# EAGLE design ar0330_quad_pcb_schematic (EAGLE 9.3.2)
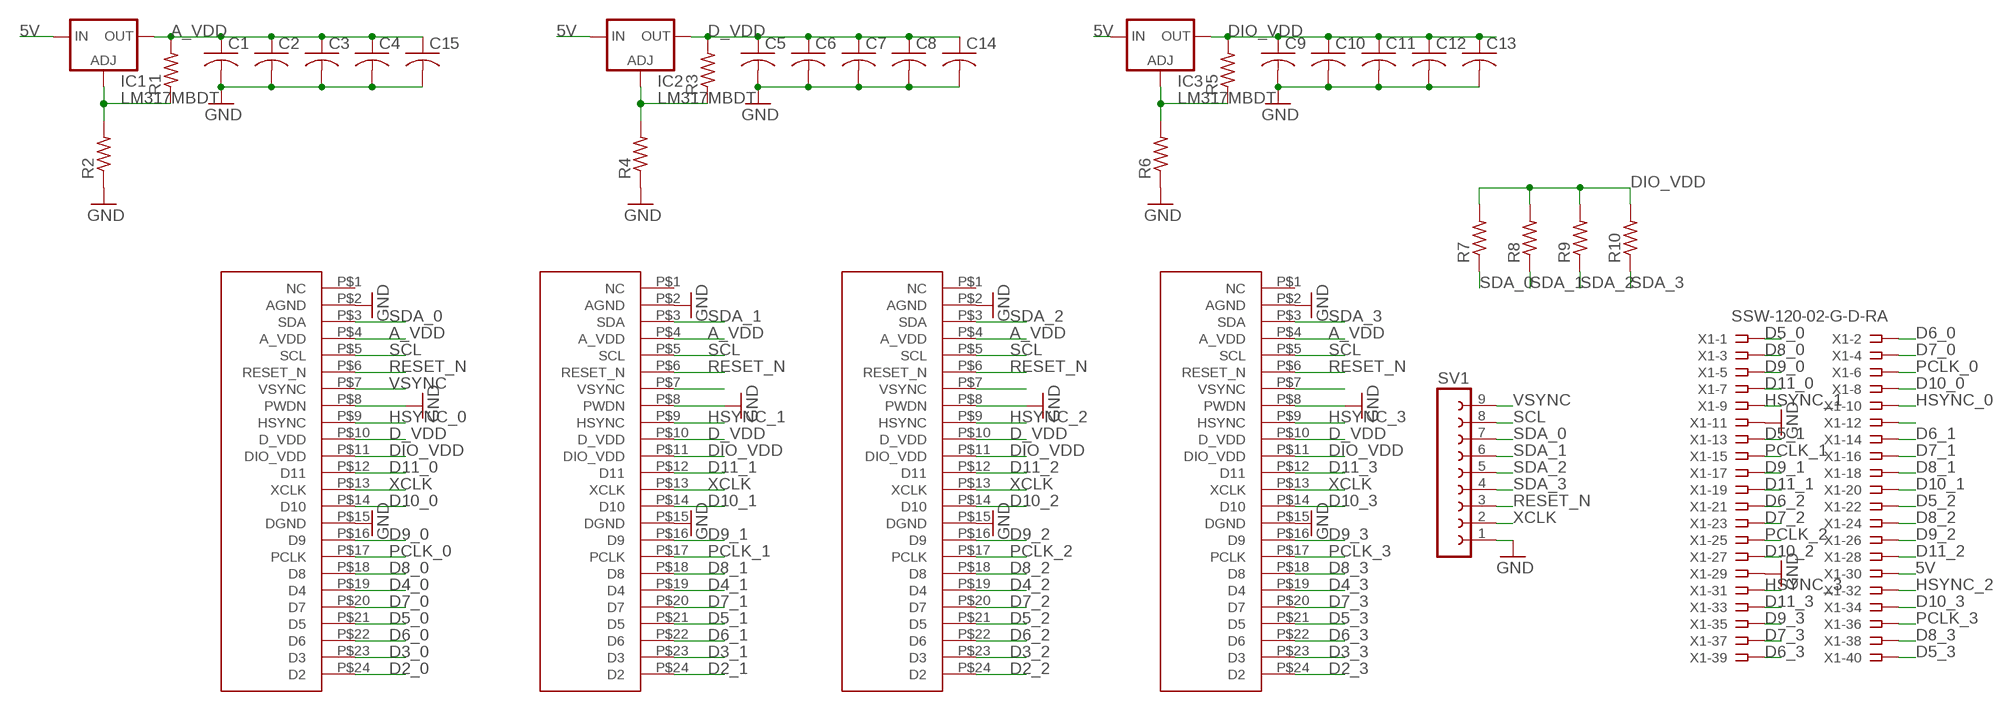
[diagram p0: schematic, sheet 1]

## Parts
C1  C-USC0805  [C0805]
C2  C-USC0805  [C0805]
C3  C-USC0805  [C0805]
C4  C-USC0805  [C0805]
C5  C-USC0805  [C0805]
C6  C-USC0805  [C0805]
C7  C-USC0805  [C0805]
C8  C-USC0805  [C0805]
C9  C-USC0805  [C0805]
C10  C-USC0805  [C0805]
C11  C-USC0805  [C0805]
C12  C-USC0805  [C0805]
C13  C-USC0805  [C0805]
C14  C-USC0805  [C0805]
C15  C-USC0805  [C0805]
IC1  LM317MBDT  [DPACK]
IC2  LM317MBDT  [DPACK]
IC3  LM317MBDT  [DPACK]
R1  R-US_R0805  [R0805]
R2  R-US_R0805  [R0805]
R3  R-US_R0805  [R0805]
R4  R-US_R0805  [R0805]
R5  R-US_R0805  [R0805]
R6  R-US_R0805  [R0805]
R7  R-US_R0805  [R0805]
R8  R-US_R0805  [R0805]
R9  R-US_R0805  [R0805]
R10  R-US_R0805  [R0805]
SV1  FE09-1  [FE09]
U$1  AR0330_FPC_24  [FPC_24_0P5]
U$2  AR0330_FPC_24  [FPC_24_0P5]
U$3  AR0330_FPC_24  [FPC_24_0P5]
U$4  AR0330_FPC_24  [FPC_24_0P5]
X1  SSW-120-02-G-D-RA  [SSW-120-02-G-D-RA]

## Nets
5V: IC1.3(IN) IC2.3(IN) IC3.3(IN) X1.30
A_VDD: C1.1 C2.1 C3.1 C4.1 C15.1 IC1.4(OUT) R1.2 U$1.P$4(A_VDD) U$2.P$4(A_VDD) U$3.P$4(A_VDD) U$4.P$4(A_VDD)
D2_0: U$1.P$24(D2)
D2_1: U$2.P$24(D2)
D2_2: U$3.P$24(D2)
D2_3: U$4.P$24(D2)
D3_0: U$1.P$23(D3)
D3_1: U$2.P$23(D3)
D3_2: U$3.P$23(D3)
D3_3: U$4.P$23(D3)
D4_0: U$1.P$19(D4)
D4_1: U$2.P$19(D4)
D4_2: U$3.P$19(D4)
D4_3: U$4.P$19(D4)
D5_0: U$1.P$21(D5) X1.1
D5_1: U$2.P$21(D5) X1.13
D5_2: U$3.P$21(D5) X1.22
D5_3: U$4.P$21(D5) X1.40
D6_0: U$1.P$22(D6) X1.2
D6_1: U$2.P$22(D6) X1.14
D6_2: U$3.P$22(D6) X1.21
D6_3: U$4.P$22(D6) X1.39
D7_0: U$1.P$20(D7) X1.4
D7_1: U$2.P$20(D7) X1.16
D7_2: U$3.P$20(D7) X1.23
D7_3: U$4.P$20(D7) X1.37
D8_0: U$1.P$18(D8) X1.3
D8_1: U$2.P$18(D8) X1.18
D8_2: U$3.P$18(D8) X1.24
D8_3: U$4.P$18(D8) X1.38
D9_0: U$1.P$16(D9) X1.5
D9_1: U$2.P$16(D9) X1.17
D9_2: U$3.P$16(D9) X1.26
D9_3: U$4.P$16(D9) X1.35
D10_0: U$1.P$14(D10) X1.8
D10_1: U$2.P$14(D10) X1.20
D10_2: U$3.P$14(D10) X1.27
D10_3: U$4.P$14(D10) X1.34
D11_0: U$1.P$12(D11) X1.7
D11_1: U$2.P$12(D11) X1.19
D11_2: U$3.P$12(D11) X1.28
D11_3: U$4.P$12(D11) X1.33
D_VDD: C5.1 C6.1 C7.1 C8.1 C14.1 IC2.4(OUT) R3.2 U$1.P$10(D_VDD) U$2.P$10(D_VDD) U$3.P$10(D_VDD) U$4.P$10(D_VDD)
DIO_VDD: C9.1 C10.1 C11.1 C12.1 C13.1 IC3.4(OUT) R5.2 R7.2 R8.2 R9.2 R10.2 U$1.P$11(DIO_VDD) U$2.P$11(DIO_VDD) U$3.P$11(DIO_VDD) U$4.P$11(DIO_VDD)
GND: C1.2 C2.2 C3.2 C4.2 C5.2 C6.2 C7.2 C8.2 C9.2 C10.2 C11.2 C12.2 C13.2 C14.2 C15.2 R2.1 R4.1 R6.1 SV1.1 U$1.P$2(AGND) U$1.P$8(PWDN) U$1.P$15(DGND) U$2.P$2(AGND) U$2.P$8(PWDN) U$2.P$15(DGND) U$3.P$2(AGND) U$3.P$8(PWDN) U$3.P$15(DGND) U$4.P$2(AGND) U$4.P$8(PWDN) U$4.P$15(DGND) X1.11 X1.29
HSYNC_0: U$1.P$9(HSYNC) X1.10
HSYNC_1: U$2.P$9(HSYNC) X1.9
HSYNC_2: U$3.P$9(HSYNC) X1.32
HSYNC_3: U$4.P$9(HSYNC) X1.31
N$16: U$2.P$7(VSYNC)
N$31: U$3.P$7(VSYNC)
N$37: X1.12
N$46: U$4.P$7(VSYNC)
N$63: IC1.1(ADJ) R1.1 R2.2
N$64: IC2.1(ADJ) R3.1 R4.2
N$66: IC3.1(ADJ) R5.1 R6.2
PCLK_0: U$1.P$17(PCLK) X1.6
PCLK_1: U$2.P$17(PCLK) X1.15
PCLK_2: U$3.P$17(PCLK) X1.25
PCLK_3: U$4.P$17(PCLK) X1.36
RESET_N: SV1.3 U$1.P$6(RESET_N) U$2.P$6(RESET_N) U$3.P$6(RESET_N) U$4.P$6(RESET_N)
SCL: SV1.8 U$1.P$5(SCL) U$2.P$5(SCL) U$3.P$5(SCL) U$4.P$5(SCL)
SDA_0: R7.1 SV1.7 U$1.P$3(SDA)
SDA_1: R8.1 SV1.6 U$2.P$3(SDA)
SDA_2: R9.1 SV1.5 U$3.P$3(SDA)
SDA_3: R10.1 SV1.4 U$4.P$3(SDA)
VSYNC: SV1.9 U$1.P$7(VSYNC)
XCLK: SV1.2 U$1.P$13(XCLK) U$2.P$13(XCLK) U$3.P$13(XCLK) U$4.P$13(XCLK)
Unconnected: U$1.P$1(NC) U$2.P$1(NC) U$3.P$1(NC) U$4.P$1(NC)

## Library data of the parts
C1-C15 = rcl:C-US: CAPACITOR, American symbol; SPICEPREFIX: C
IC1-IC3 = v-reg:LM317?*: 500 mA Adjustable Output Positive Voltage Regulator Source: http://www.onsemi.co.jp .. LM317M-D.PDF
R1-R10 = rcl:R-US_: RESISTOR, American symbol; SPICEPREFIX: R
SV1 = con-lsta:FE09-1: FEMALE HEADER; OC_FARNELL: unknown; OC_NEWARK: unknown
U$1-U$4 = FPC_24_0P5:AR0330_FPC_24
X1 = con-samtec:SSW-120-02-G: THROUGH-HOLE .025" SQ POST SOCKET Source: Samtec SSW.pdf; MF: Samtec Inc.; MPN: SSW-120-02-G-D-RA; OC_FARNELL: unknown; OC_NEWARK: 11P9640

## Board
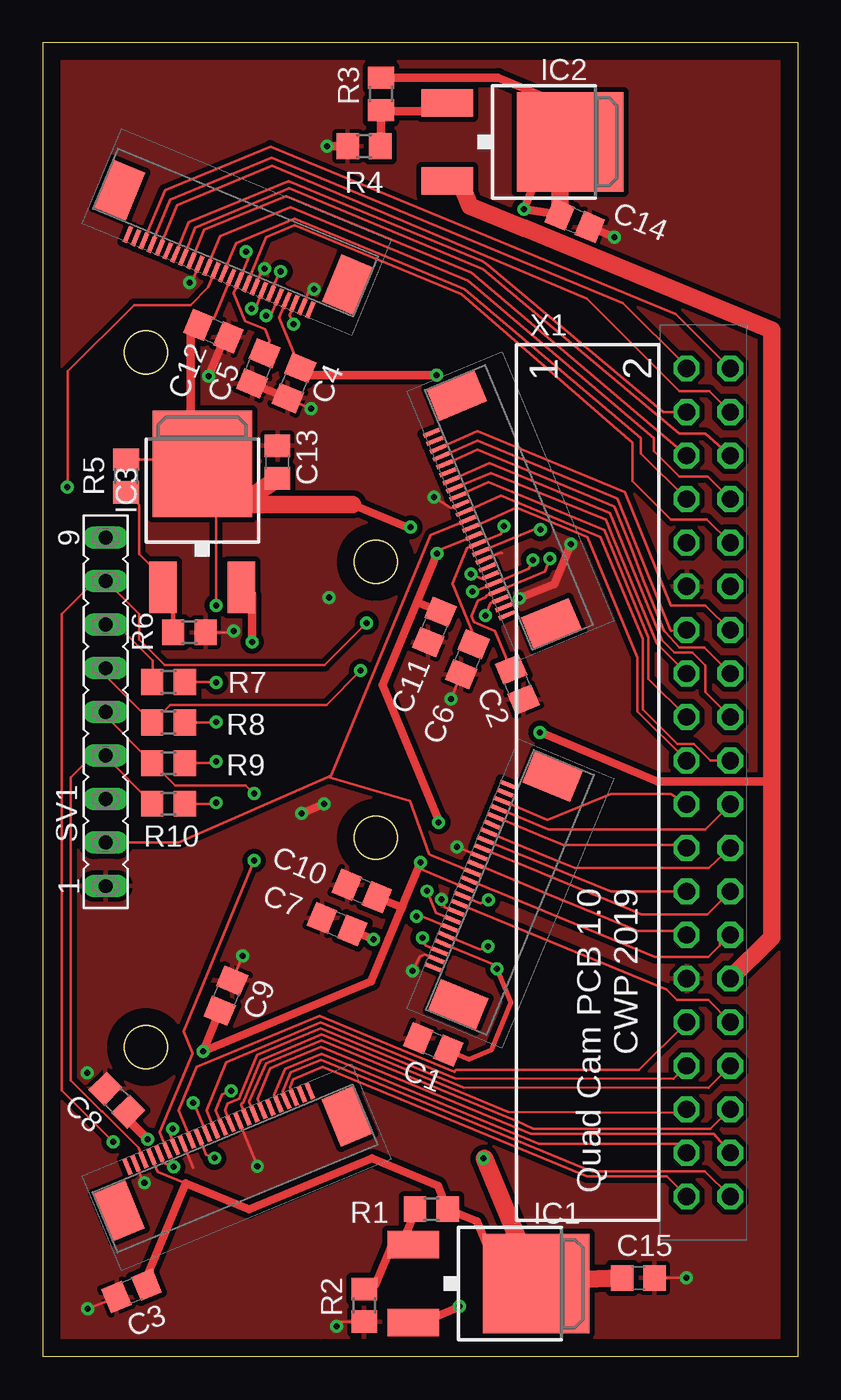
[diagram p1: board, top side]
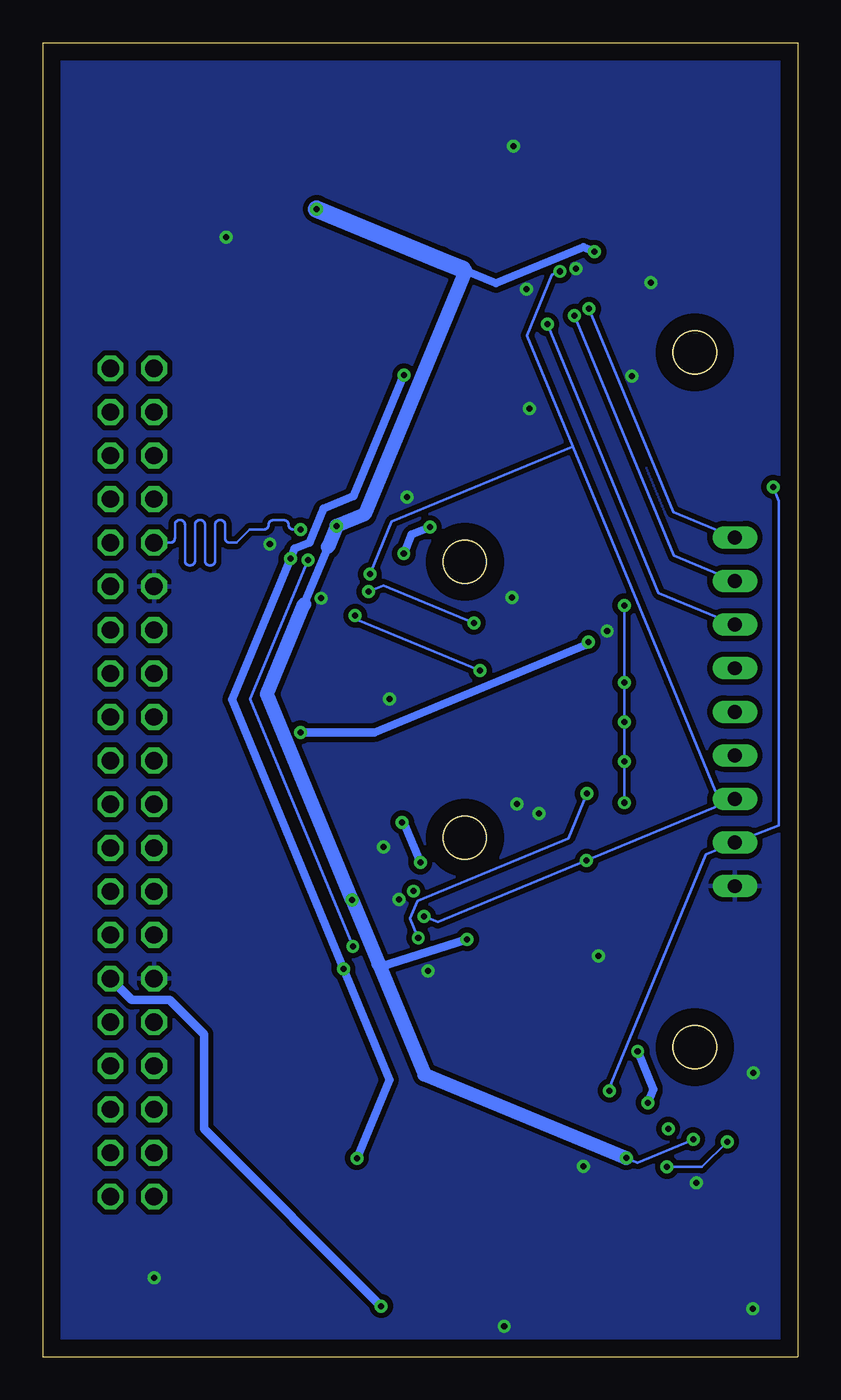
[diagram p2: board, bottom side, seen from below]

Size 44 x 76.56 mm. Coordinates in mm from the lower left corner, seen from the top.
Outline: 44,76.56 0,76.56 0,0 44,0 44,76.56
Outline: circle at 19.4,30.24 radius 1.25
Outline: circle at 19.4,46.32 radius 1.25
Outline: circle at 19.4,30.24 radius 1.25
Outline: circle at 19.4,46.32 radius 1.25
Outline: circle at 6,18.03 radius 1.25
Outline: circle at 6,58.52 radius 1.25
Copper layers (1*16): Top 0.035mm / dielectric 1.5mm / Bottom 0.035mm
Design rules "default": minimum track width 6mil, minimum drill 0.35mm, track to track 6mil, track to pad 6mil, pad to pad 6mil, via to via 6mil, smd to smd 6mil, copper to edge 40mil, drill to drill 6mil, minimum pad ring 10mil, minimum via ring 8mil, stop-mask expansion 4mil, vias tented up to drill 0mil, thermal gap 10mil
Holes 2.5 mm at 6,58.52 19.4,46.32 19.4,30.24 6,18.03

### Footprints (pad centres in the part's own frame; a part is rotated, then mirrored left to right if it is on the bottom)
C0805 = smd 1.3 x 1.5: 1 -0.95,0; 2 0.95,0
DPACK = smd 1.6 x 3: 1 -2.28,-4.8; 3 2.28,-4.8 | smd 5.8 x 6.2: 4 0,2.38
R0805 = smd 1.3 x 1.5: 1 -0.95,0; 2 0.95,0
FE09 = drill 0.813 long: 1 -10.16,0; 2 -7.62,0; 3 -5.08,0; 4 -2.54,0; 5 0,0; 6 2.54,0; 7 5.08,0; 8 7.62,0; 9 10.16,0
FPC_24_0P5 = smd 0.25 x 1: P$1 -5.75,0.6; P$2 -5.25,0.6; P$3 -4.75,0.6; P$4 -4.25,0.6; P$5 -3.75,0.6; P$6 -3.25,0.6; P$7 -2.75,0.6; P$8 -2.25,0.6; P$9 -1.75,0.6; P$10 -1.25,0.6; P$11 -0.75,0.6; P$12 -0.25,0.6; P$13 0.25,0.6; P$14 0.75,0.6; P$15 1.25,0.6; P$16 1.75,0.6; P$17 2.25,0.6; P$18 2.75,0.6; P$19 3.25,0.6; P$20 3.75,0.6; P$21 4.25,0.6; P$22 4.75,0.6; P$23 5.25,0.6; P$24 5.75,0.6 | smd 2 x 3: P$25 -7.2,-1.6; P$26 7.2,-1.6
SSW-120-02-G-D-RA = drill 1 pad 1.5 octagon: 1 -24.13,1.524; 2 -24.13,4.064; 3 -21.59,1.524; 4 -21.59,4.064; 5 -19.05,1.524; 6 -19.05,4.064; 7 -16.51,1.524; 8 -16.51,4.064; 9 -13.97,1.524; 10 -13.97,4.064; 11 -11.43,1.524; 12 -11.43,4.064; 13 -8.89,1.524; 14 -8.89,4.064; 15 -6.35,1.524; 16 -6.35,4.064; 17 -3.81,1.524; 18 -3.81,4.064; 19 -1.27,1.524; 20 -1.27,4.064; 21 1.27,1.524; 22 1.27,4.064; 23 3.81,1.524; 24 3.81,4.064; 25 6.35,1.524; 26 6.35,4.064; 27 8.89,1.524; 28 8.89,4.064; 29 11.43,1.524; 30 11.43,4.064; 31 13.97,1.524; 32 13.97,4.064; 33 16.51,1.524; 34 16.51,4.064; 35 19.05,1.524; 36 19.05,4.064; 37 21.59,1.524; 38 21.59,4.064; 39 24.13,1.524; 40 24.13,4.064

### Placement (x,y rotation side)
C1  22.76,18.19 157.5 top
C2  27.65,39.16 292.5 top
C3  5.17,3.83 202.5 top
C4  14.64,56.73 247.5 top
C5  12.56,57.59 247.5 top
C6  24.75,40.64 247.5 top
C7  17.14,25.2 157.5 top
C8  4.31,14.94 135 top
C9  10.67,21.03 67.5 top
C10  18.6,27.14 157.5 top
C11  22.82,42.52 247.5 top
C12  9.94,59.76 337.5 top
C13  13.67,52.13 90 top
C14  31,66.19 337.5 top
C15  34.71,4.58 0 top
IC1  26.38,4.25 270 top
IC2  28.36,70.79 270 top
IC3  9.29,49.64 0 top
R1  22.64,8.59 0 top
R2  18.73,2.98 90 top
R3  19.71,73.58 90 top
R4  18.72,70.54 0 top
R5  4.86,51.33 90 top
R6  8.54,42.21 180 top
R7  7.32,39.31 0 top
R8  7.32,36.95 0 top
R9  7.32,34.58 0 top
R10  7.32,32.22 0 top
SV1  3.66,37.58 90 top
U$1  10.51,63.75 157.5 top
U$2  25.4,48.76 112.5 top
U$3  25.48,27.78 67.5 top
U$4  10.48,12.72 22.5 top
X1  36,33.46 270 top

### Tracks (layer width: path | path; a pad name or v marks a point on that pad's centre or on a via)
5V  (via drill 0.35)
  Top 0.508: v24.29,2.94 24.29,2.89 22.08,1.97 IC1.3 | v12.19,41.65 12.19,44.35 12.06,44.67 11.74,44.67 IC3.3 | 42.48,33.78 42.23,33.53 35.83,33.53 29.04,36.38 v28.98,36.38
  Top 1.016: IC2.3 23.83,68.62 24.34,68.41 24.9,67.05 28.04,65.75 28.09,65.77 42.48,59.81 42.48,33.78 42.48,24.44 X1.30
  Bottom 0.508: v28.98,36.38 24.66,36.38 12.36,41.48 v12.19,41.65 | v24.29,2.94 34.61,13.27 34.61,18.78 36.61,20.78 38.81,20.78 X1.30
A_VDD  (via drill 0.35)
  Top 0.152: U$1.P$4 13.78,60.55 C4.1 15.42,57.19 | U$4.P$4 6.68,10.78 8.31,10.1 | U$3.P$4 26.4,22.8 v26.48,22.6 | v29.56,46.5 29.25,45.75 U$2.P$4 25.85,44.34 25.82,44.25 25.35,44.06 24.98,43.17 25.14,42.8 26.36,42.29 C2.1
  Top 0.254: C1.1 24.83,17.33 26.14,17.87 27.29,20.64 v26.48,22.6
  Top 0.508: 28.7,4.39 IC1.4 26.4,5.23 25.3,7.89 R1.2 23.03,9.96 19.19,11.55 12.01,8.57 8.31,10.1 5.95,4.42 C3.1 | 25.74,11.54 v25.69,11.56 | v22.95,57.19 15.42,57.19
  Top 1.016: 25.74,11.54 28.7,4.39 C15.1
  Bottom 0.508: v25.69,11.56 23.8,16.14 v26.48,22.6 32.97,38.28 v29.56,46.5 29.32,47.1 28.45,47.45 27.64,49.41 25.89,50.14 22.98,57.18 v22.95,57.19
D4_2
  Top 0.152: U$3.P$19 26.21,31.01
D5_0
  Top 0.152: U$1.P$21 7.43,67.42 13.34,69.87 33.82,61.39 37.52,57.69 X1.1
D5_1
  Top 0.152: U$2.P$21 25.33,53.39 33.5,50 36.58,42.34 36.63,42.29 X1.13
D5_2
  Top 0.152: U$3.P$21 29.46,30.73 38.6,30.73 X1.22
D5_3
  Top 0.152: U$4.P$21 13.96,15.43 14.43,16.57 16.2,17.31 31.97,10.8 38.6,10.8 X1.40
D6_0
  Top 0.152: U$1.P$22 7.12,67.97 13.26,70.52 36.04,61.11 36.9,60.75 X1.2
D6_1
  Top 0.152: U$2.P$22 25.33,53.93 33.92,50.37 36.61,43.78 38.61,43.78 X1.14
D6_2
  Top 0.152: U$3.P$22 29.41,31.28 33.11,32.78 36.61,32.78 X1.21
D6_3
  Top 0.152: U$4.P$22 14.39,15.68 14.59,16.16 16.31,16.87 31.72,10.49 36.36,10.49 X1.39
D7_0
  Top 0.152: U$1.P$20 7.84,67.1 13.36,69.39 31.72,61.67 37.11,56.28 38.83,56.28 X1.4
D7_1
  Top 0.152: U$2.P$20 25.33,52.84 33.3,49.54 34.25,47.25 34.98,45.31 36.2,42.31 36.24,42.27 36.24,42.26 37.09,41.33 38.56,41.33 X1.16
D7_2
  Top 0.152: U$3.P$20 29.13,30.33 30.34,29.83 37.35,29.83 X1.23
D7_3
  Top 0.152: U$4.P$20 13.48,15.27 14.11,16.77 16.25,17.66 28.92,12.41 36.98,12.41 X1.37
D8_0
  Top 0.152: U$1.P$18 8.5,66.1 14.32,68.51 25.63,63.83 25.95,63.59 36.16,55.03 X1.3
D8_1
  Top 0.152: U$2.P$18 26.02,52.08 33.05,49.17 36.07,41.76 36.81,41.02 37.08,41.02 37.2,41.02 37.21,41.02 37.86,41.02 38.61,40.28 38.61,38.72 X1.18
D8_2
  Top 0.152: U$3.P$18 29.7,29.01 31.01,28.48 38.81,28.48 X1.24
D8_3
  Top 0.152: U$4.P$18 12.51,15.01 13.25,16.81 14.23,17.22 16.2,18.05 28.43,12.98 39.11,12.98 X1.38
D9_0
  Top 0.152: U$1.P$16 9.41,65.66 14.17,67.64 24.99,63.16 X1.5
D9_1
  Top 0.152: U$2.P$16 25.98,50.95 32.73,48.15 35.3,41.91 35.3,39.49 X1.17
D9_2
  Top 0.152: U$3.P$16 25.61,29.61 28.78,28.3 29.07,28.19 34.22,26.05 34.88,25.78 38.73,25.78 X1.26
D9_3
  Top 0.152: U$4.P$16 11.56,14.68 11.6,14.77 11.67,14.8 12.69,17.28 16.25,18.77 25.93,14.76 27.12,14.27 37.33,14.21 X1.35
D10_0
  Top 0.152: U$1.P$14 10.33,65.28 14.45,66.99 24.79,62.7 35.61,53.53 35.61,52.78 37.11,51.28 38.75,51.28 X1.8
D10_1
  Top 0.152: U$2.P$14 26.69,50.17 32.51,47.76 34.97,41.81 34.97,40.76 34.98,40.76 34.98,37.7 36.97,35.71 37.93,35.71 38.91,34.73 X1.20
D10_2
  Top 0.152: U$3.P$14 25.24,28.7 29.47,26.95 34.39,24.91 34.62,24.81 34.71,24.82 37.27,24.82 X1.27
D10_3
  Top 0.152: U$4.P$14 10.61,14.36 10.78,14.76 11.43,15.03 11.53,15.26 | 11.53,15.26 | 11.53,15.26 12.49,17.57 16.18,19.14 24.5,15.69 38.78,15.66 X1.34
D11_0
  Top 0.152: U$1.P$12 11.25,64.9 14.67,66.31 24.15,62.39 24.58,62.21 34.86,53.53 34.86,52.63 X1.7
D11_1
  Top 0.152: U$2.P$12 27.61,49.47 31.75,47.75 34.65,40.75 34.65,37.6 X1.19
D11_2
  Top 0.152: X1.28 39.52,24.61 39.47,23.98 38.77,23.28 35.66,23.28 26.23,27.19 26.22,27.21 26.2,27.21 U$3.P$12
D11_3
  Top 0.152: U$4.P$12 9.53,14.36 10.69,17.16 16.18,19.48 24.03,16.22 36.76,16.19 X1.33
D_VDD  (via drill 0.35)
  Top 0.152: C5.1 13.23,59.21 12.96,59.86 11.8,60.34 11.12,61.98 U$1.P$10 11.99,64.05 v11.85,64.38 | v26.88,48.41 26.69,47.93 U$2.P$10 24.73,47.12 23.87,45.06 25.22,41.79 C6.1 | U$3.P$10 25.51,26.41 v25.97,26.6 | U$4.P$10 9.52,11.77 v10,11.57 | C7.1 18.03,24.84
  Top 0.508: R3.2 26.54,74.53 30.06,73.07 30.87,71.11 IC2.4 29.44,70.25 v28.04,66.88 C14.1 | 18.03,24.84 v19.27,24.32 | C8.1 4.98,14.17 5.24,13.53 v6.1,12.67
  Top 1.016: C14.1 30.12,69.29
  Bottom 0.152: v6.1,12.67 6.11,12.64 9.35,11.3 v10,11.57
  Bottom 0.508: 19.54,63.36 19.38,63.29 17.59,62.55 12.5,64.65 v11.85,64.38 | 27.39,47.19 28.77,43.85 | v19.27,24.32 24.35,22.7 24.44,22.91
  Bottom 0.813: 19.38,63.29 25.27,49.08 v26.88,48.41 | 30.94,38.61 v25.97,26.6 24.44,22.91 21.76,16.44 v10,11.57 | 30.94,38.61 | 30.94,38.61 28.77,43.85 | v26.88,48.41 | v26.88,48.41 27.39,47.19
  Bottom 1.016: v28.04,66.88 20.85,63.9 19.54,63.36
DIO_VDD  (via drill 0.35)
  Top 0.152: U$2.P$11 23.04,46.96 v22.96,46.79 | U$3.P$11 22.01,28.41 21.93,28.6 v22,28.79 | U$4.P$11 8.8,14.82 v8.75,14.79 | C12.1 9.97,60.5 U$1.P$11 | R10.2 10.05,32.22 v10.11,32.28 | R9.2 10.01,34.58 v10.11,34.68 | R8.2 10.08,36.95 v10.11,36.98 | R7.2 10.07,39.31 v10.11,39.28 | v10.11,43.78 10.11,50.78 10.45,51.12 | R5.2 9.18,52.27 9.28,52.17 IC3.4 9.28,52.78 9.28,54.16
  Top 0.508: 18.06,49.65 21.34,48.29 v21.44,48.33 | v22.96,46.79 21.8,43.97 | C11.1 21.8,43.97 | 21.8,43.97 19.8,39.14 23.06,31.26 v23.06,31.14 | v22,28.79 20.97,26.3 20.92,26.17 | 20.92,26.17 20.85,26.01 19.13,21.86 v9.33,17.8 C9.1 | C10.1 20.92,26.17 | C12.1 8.61,59.67 8.61,53.45 9.28,52.78
  Top 1.016: IC3.4 9.65,51.92 10.45,51.12 11.74,49.83 | C13.1 11.74,49.83 | 18.06,49.65 11.92,49.65 11.74,49.83
  Bottom 0.152: v10.11,32.28 v10.11,34.68 v10.11,36.98 v10.11,39.28 v10.11,43.78
  Bottom 0.508: v21.44,48.33 22.51,47.89 v22.96,46.79 | v23.06,31.14 22.99,31.17 v22,28.79 | v9.33,17.8 8.42,15.59 v8.75,14.79
GND  (via drill 0.35)
  Top 0.152: U$1.P$2 15.49,62.06 v15.82,62.2 | U$1.P$15 8.69,62.64 v8.57,62.59 | U$3.P$2 22.26,23.43 21.97,23.31 v21.55,22.48 | U$3.P$15 v24.13,29.69 | U$2.P$2 27.72,44.03 v27.78,44.19 | U$4.P$15 12.51,11.09 v12.5,11.07 | U$4.P$2 5.86,10.16 v5.92,10.14 | U$3.P$8 23.44,26.19 v23.25,26.65 | U$1.P$8 12.76,63.32 v12.94,63.39 | U$2.P$8 26.71,46.86 26.77,46.83 | U$4.P$8 8.76,11 | C4.2 14.3,55.79 v15.64,55.23 | C9.2 v11.63,23.34 | C6.2 v23.79,38.33 | U$2.P$15 23.79,49.45 v22.79,50.08 | R6.1 11.04,42.21 v11.11,42.28 | C3.2 v2.61,2.78 | R2.1 17.37,2.03 v17.11,1.78 | v37.51,4.58 C15.2
  Top 0.508: C4.2 C5.2 | C12.2 10.46,59.04 v9.66,57.13 | C14.2 v33.31,65.23 | v16.57,70.54 R4.1 | v27.78,44.19 29.81,45.03 v30.77,47.34 | v15.07,31.66 v16.38,32.2
  other vias: 16.67,44.24 2.59,16.54
  pour Top (isolate 0.305): 0.21,76.78 43.94,76.52 44.22,0.1 0.29,-0.11
  pour Bottom (isolate 0.305): 0.02,76.32 43.94,76.52 43.75,0.29 0.29,-0.11
HSYNC_0
  Top 0.152: U$1.P$9 13.02,65.25 14.68,65.94 24.41,61.91 34.36,53.28 34.36,51.03 36.61,48.78 38.71,48.78 X1.10
HSYNC_1  (via drill 0.35)
  Top 0.152: U$2.P$9 28.82,48.28 v28.99,48.2
  Bottom 0.152: v28.99,48.2 29.41,48.2 arc90 29.68,48.47 arc-90 29.95,48.74 30.58,48.74 arc-90 30.84,48.47 arc90 31.11,48.2 31.95,48.2 32.72,47.43 33.11,47.43 arc90 33.38,47.7 33.38,48.48 arc-90 33.64,48.75 33.7,48.75 arc-90 33.96,48.48 33.96,46.38 arc90 34.23,46.11 34.28,46.11 arc90 34.55,46.38 34.55,48.48 arc-90 34.81,48.75 34.87,48.75 arc-90 35.13,48.48 35.13,46.38 arc90 35.4,46.11 35.45,46.11 arc90 35.72,46.38 35.72,48.48 arc-90 35.99,48.75 36.04,48.75 arc-90 36.3,48.48 36.3,47.7 arc90 36.57,47.43 X1.9
HSYNC_2
  Top 0.152: U$3.P$9 36.33,21.39 36.94,20.78 38.77,20.78 X1.32
HSYNC_3
  Top 0.152: U$4.P$9 7.91,14.36 8.95,16.87 16.14,19.85 23.99,16.6 24.09,16.7 34.73,16.7 X1.31
N$31  (via drill 0.35)
  Top 0.152: v22.4,27.12 22.59,26.65 22.91,25.86 U$3.P$7
N$46  (via drill 0.35)
  Top 0.152: U$4.P$7 7.41,12.94 v7.55,13.28
N$63
  Top 0.508: R2.2 19.4,4.21 20.43,6.71 20.8,6.86 IC1.1 21.24,7.35 21.66,8.36 21.63,8.44 R1.1
N$64
  Top 0.508: R4.2 19.67,70.52 19.71,70.43 R3.1 19.77,72.57 23.06,72.57 IC2.1
N$66
  Top 0.152: IC3.1 7,45.38 5.61,46.78 5.61,49.62 R5.1
  Top 0.254: R6.2 7.59,43.26 IC3.1 7,45.89
PCLK_0
  Top 0.152: U$1.P$17 8.86,65.78 14.04,67.95 14.34,68.08 25.65,63.37 37.11,53.78 38.61,53.78 X1.6
PCLK_1
  Top 0.152: X1.15 35.9,41.43 35.87,41.44 35.86,41.47 35.79,41.55 33.2,47.82 32.81,48.78 26.11,51.48 U$2.P$17
PCLK_2
  Top 0.152: U$3.P$17 33.11,27.11 X1.25
PCLK_3
  Top 0.152: U$4.P$17 12.02,14.85 12.03,14.87 13.01,17.08 13.14,17.13 16.25,18.44 27.01,13.98 27.59,13.73 28.6,13.28 38.91,13.28 X1.36
RESET_N  (via drill 0.35)
  Top 0.152: U$1.P$6 13.8,63.22 v13.86,63.24 | U$3.P$6 21.95,25.72 v21.77,25.65 | U$4.P$6 6.81,13.08 8.72,17.68 8.19,18.96 v12.31,28.91 | v24.94,45.6 25.61,45.32 U$2.P$6
  Bottom 0.152: v13.86,63.24 14.31,63.05 15.78,59.5 13.1,53.04 | 13.1,53.04 7.44,39.35 | 7.44,39.35 4.79,32.96 SV1.3 v12.31,28.91 20.98,25.32 v21.77,25.65 | 13.1,53.04 23.68,48.66 v24.94,45.6 | 7.44,39.35
SCL  (via drill 0.35)
  Top 0.152: U$1.P$5 13.34,60.79 v13.01,60.65 | v25.03,44.58 25.08,44.56 U$2.P$5 28.34,45.91 v28.56,46.43 | U$3.P$5 25.48,23.72 v25.94,23.91 | v7.62,11.05 7.01,11.3 U$4.P$5 | v4.11,12.53 1.11,15.53 1.11,43.28 3.03,45.19 SV1.8 3.66,45.22 3.66,45.23 5.61,43.28 5.61,41.78 7.1,40.29 16.41,40.29 v18.88,42.76
  Bottom 0.152: v13.01,60.65 7.22,46.67 SV1.8 | v18.88,42.76 24.16,44.94 v25.03,44.58 | v25.94,23.91 31.91,38.33 v28.56,46.43 | v4.11,12.53 5.59,11.05 v7.62,11.05
SDA_0  (via drill 0.35)
  Top 0.152: U$1.P$3 14.38,60.69 v14.6,60.16 | SV1.7 4.3,42.65 6.39,40.56 6.39,39.33 R7.1
  Bottom 0.152: v14.6,60.16 8.11,44.5 SV1.7
SDA_1  (via drill 0.35)
  Top 0.152: v18.52,39.97 16.53,37.99 7.41,37.99 R8.1 3.66,39.66 SV1.6 | v25.8,43.18 26.1,43.9 U$2.P$3
  Bottom 0.152: v18.52,39.97 25.7,42.95 v25.8,43.18
SDA_2  (via drill 0.35)
  Top 0.152: U$3.P$3 22.31,23.95 v22.12,24.41 | SV1.5 3.66,37.33 R9.1 7.71,33.28 11.83,33.28 v12.3,32.8
  Bottom 0.152: v12.3,32.8 13.38,30.2 22.16,26.56 22.59,25.54 v22.12,24.41
SDA_3
  Top 0.152: U$4.P$3 5.57,12.15 3.45,14.28 3.44,14.28 1.62,16.1 1.62,33.74 2.92,35.03 SV1.4 3.66,35 R10.1
VSYNC  (via drill 0.35)
  Top 0.152: U$1.P$7 12.41,61.17 v12.16,61.06
  Bottom 0.152: SV1.9 7.25,49.22 v12.16,61.06
XCLK  (via drill 0.35)
  Top 0.152: U$3.P$13 22.6,29.24 22.5,29.28 21.41,32.38 16.61,33.78 | U$2.P$13 22.6,47.86 16.82,33.91 16.8,33.87 16.61,33.78 | SV1.2 7.91,29.95 16.61,33.78 | U$4.P$13 10.07,14.36 10.46,15.28 v10.97,15.5 | U$1.P$13 9.64,62.32 8.6,61.28 5.31,61.28 1.45,57.42 1.45,50.7 v1.43,50.68
  Bottom 0.152: v10.97,15.5 11.01,15.6 5.35,29.25 SV1.2 1.09,30.95 1.09,49.87 v1.43,50.68

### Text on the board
tNames: Quad Cam PCB 1.0 / CWP 2019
